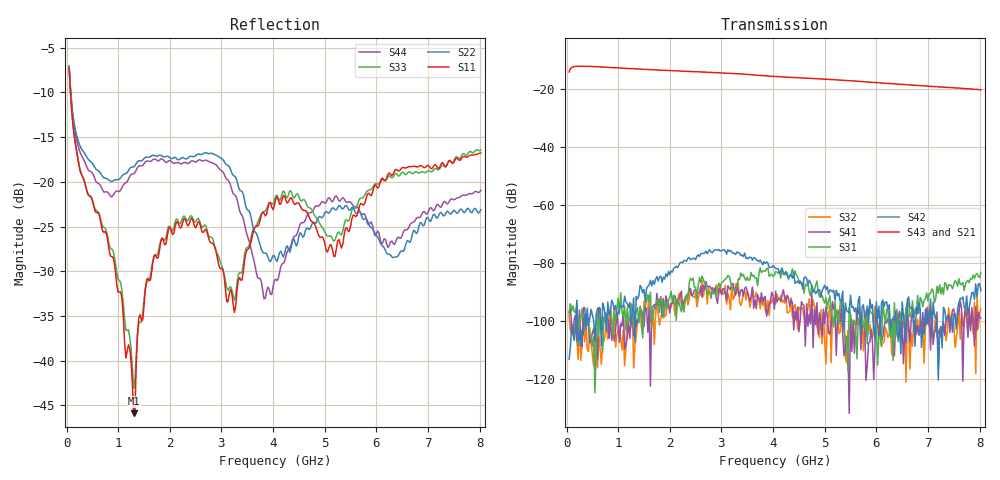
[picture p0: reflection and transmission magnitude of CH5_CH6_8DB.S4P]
!Agilent Technologies,E5071C,MY46316741,A.11.02
!Date: Mon Jun 01 10:40:58 2026
!Data & Calibration Information:
!1:CH5 INPUT 2:CH5 OUTPUT 3:CH6 INPUT 4:CH6 OUTPUT
!Freq	S11:SOLT4(ON)	S12:SOLT4(ON)	S13:SOLT4(ON)	S14:SOLT4(ON)
!	S21:SOLT4(ON)	S22:SOLT4(ON)	S23:SOLT4(ON)	S24:SOLT4(ON)
!	S31:SOLT4(ON)	S32:SOLT4(ON)	S33:SOLT4(ON)	S34:SOLT4(ON)
!	S41:SOLT4(ON)	S42:SOLT4(ON)	S43:SOLT4(ON)	S44:SOLT4(ON)
!PortZ  Port1:50+j0  Port2:50+j0  Port3:50+j0  Port4:50+j0
!Above PortZ is port z conversion or system Z0 setting when saving the data.
!When reading, reference impedance value at option line is always used.
# Hz S dB R 50
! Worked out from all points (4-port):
!   320 points, 50 MHz to 8.025 GHz, reference 50 ohm
!   strongest paths, dB at 50 MHz, 2.05 GHz, 4.05 GHz, 6.05 GHz, 8.025 GHz:
!     S43: -14.2, -13.8, -15.8, -17.9, -20.3
!     S21: -14.2, -13.9, -16.0, -18.1, -20.6
!     S42: -113.2, -83.1, -81.8, -94.9, -89.5
!     S31: -97.8, -93.2, -83.0, -105.4, -83.3
!     S41: -97.0, -93.8, -89.7, -105.8, -99.0
!     S32: -98.2, -93.2, -94.1, -102.4, -95.7
!   lowest |S11| = -45.9 dB at 1.3 GHz (marker M1), VSWR 1.01, Z = 49.8 - j0.483 ohm
!   |S11| at or under -10 dB: 75.9 MHz to end of sweep
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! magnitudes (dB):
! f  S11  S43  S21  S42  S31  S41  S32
! 50 MHz  -7.3  -14.2  -14.2  -113.2  -97.8  -97.0  -98.2
! 425 MHz  -21.5  -12.3  -12.4  -101.2  -99.3  -101.6  -110.5
! 1.3 GHz  -45.9  -13.1  -13.2  -92.0  -102.6  -104.9  -116.2
! 2 GHz  -25.1  -13.7  -13.9  -84.1  -91.7  -97.2  -96.1
! 3.25 GHz  -34.6  -14.7  -14.9  -76.6  -89.6  -89.6  -91.7
! 3.825 GHz  -23.5  -15.5  -15.7  -79.5  -82.7  -92.1  -92.0
! 8.025 GHz  -16.8  -20.3  -20.6  -89.5  -83.3  -99.0  -95.7
